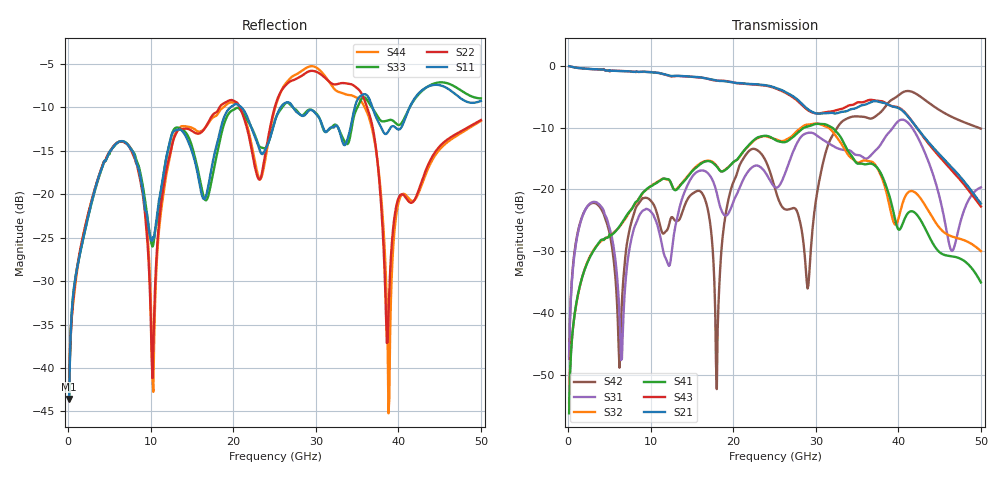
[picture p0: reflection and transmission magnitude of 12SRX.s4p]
! DAC39RF10ACK
! 256-pin FCBGA package
! Texas Instruments 8/20/2022
! Single-ended  S-parameters
! PORT#  PORT_NAME  NET_NAME
! PORT1:  xSRXN.DIEBUMP  xSRXN
! PORT2:  xSRXN.BGA  xSRXN
! PORT3:  xSRXP.DIEBUMP  xSRXP
! PORT4:  xSRXP.BGA  xSRXP
! Touchstone Ver. 1.0
! Number of ports is 4
# Hz	S	MA	R	50.000000
! SCATTERING PARAMETERS  :
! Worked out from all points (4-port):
!   500 points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, 100 MHz to 50 GHz, reference 50 ohm
!   strongest paths, dB at 100 MHz, 12.6 GHz, 25.1 GHz, 37.6 GHz, 50 GHz:
!     S21: 0.0, -1.6, -3.5, -5.8, -22.3
!     S43: 0.0, -1.7, -3.6, -5.7, -22.8
!     S41: -56.3, -19.5, -12.0, -16.8, -35.1
!     S32: -54.6, -19.5, -11.9, -16.9, -30.0
!     S31: -47.4, -29.3, -19.7, -13.2, -19.7
!     S42: -47.0, -24.5, -20.1, -7.8, -10.2
!   lowest |S11| = -43.6 dB at 100 MHz (marker M1), VSWR 1.01, Z = 50.5 + j0.443 ohm
!   |S11| at or under -10 dB: start of sweep to 19.65 GHz; 20.99 GHz to 25.73 GHz (4.744 GHz wide, 20.3 % of centre); 27.25 GHz to 34.72 GHz (7.471 GHz wide, 24.1 % of centre)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
1e8  0.006636 41.3  0.9853 -3.1  0.00429 84.0  0.001252 -95.3
     0.9947 -3.1  0.008221 23.3  0.00145 -101.8  0.004778 81.9
     0.004252 83.9  0.001868 -76.3  0.006489 40.9  0.9912 -3.4
     0.001538 -102.4  0.004473 79.2  0.9948 -3.1  0.008214 40.3
6.3e9  0.2019 -73.5  0.906 -176.6  0.006673 -130.5  0.05056 90.7
       0.9092 -176.2  0.2017 -100.3  0.05137 92.4  0.005023 153.7
       0.006527 -131.2  0.05076 91.6  0.2014 -71.9  0.9046 -175.4
       0.05119 92.1  0.005312 150.5  0.9106 -175.1  0.2015 -100.1
1.29e10  0.2326 -103.5  0.8305 0.6  0.0473 158.3  0.0993 -102.7
         0.8319 0.7  0.2154 -72.8  0.1004 -100.4  0.05696 31.2
         0.04731 157.5  0.09961 -100.9  0.2389 -100.2  0.826 2.9
         0.09871 -103.0  0.05622 32.4  0.8258 3.2  0.22 -70.4
1.92e10  0.2985 -49.3  0.7498 -174.8  0.06181 -178.5  0.1467 92.2
         0.7478 -174.7  0.3413 -123.5  0.1476 93.9  0.07139 95.3
         0.06166 -178.2  0.148 94.1  0.278 -44.9  0.7552 -171.5
         0.1467 92.3  0.07071 96.7  0.7525 -171.3  0.329 -122.2
3.56e10  0.3724 -111.2  0.4791 108.0  0.1818 -30.4  0.1609 -64.1
         0.48 107.4  0.3759 142.5  0.1673 -53.8  0.3879 70.3
         0.1843 -31.3  0.1699 -53.4  0.3571 -108.5  0.512 113.3
         0.1614 -64.8  0.3881 70.4  0.5067 113.0  0.3376 148.1
3.88e10  0.2312 -114.0  0.4839 5.9  0.2808 134.4  0.09391 -171.4
         0.4846 6.1  0.01975 -66.8  0.08027 -160.3  0.5039 54.5
         0.2859 134.4  0.08045 -161.3  0.2667 -117.4  0.4903 13.4
         0.09363 -170.4  0.504 54.4  0.4846 13.5  0.005488 44.2
5e10  0.3445 -121.4  0.06852 99.3  0.09516 -1.8  0.03109 -11.1
      0.07669 114.6  0.2673 -122.3  0.01806 30.2  0.3217 -32.3
      0.1039 -2.1  0.03168 -5.2  0.3561 -131.6  0.0701 110.4
      0.01766 13.0  0.3105 -33.0  0.07276 128.5  0.2647 -120.6
